| TEXAS INSTRUMENTS INCORPORATED
| Standard Linear and Logic Group
| IBIS Model of SN74LVCHR16245A
| 16-BIT BUS TRANSCEIVER WITH 3-STATE OUTPUTS
| This file contains package information for the following:
|  SSOP 48-pin (DL) package as [Component] LVCHR16245A_DL
|  TSSOP 48-pin (DGG) package as [Component] LVCHR16245A_DGG
|  VFBGA 48-pin (GQL) package as [Component] LVCHR16245A_GQL
| This device can be powered at the following Vccs:
|  1.8 volt Vcc
|  2.5 volt Vcc
|  3.3 volt Vcc
| This file provides unique models under the [Model Selector] for each Vcc.
| For operation at a specific Vcc, select the appropriate model after each
| [Model Selector] keyword.
[IBIS Ver]   3.2
[Comment char]  |_char
[File Name]   sn74lvchr16245a.ibs
[File Rev]   1.2 | e_die
[Date]   January 8, 2003
[Source]   Data created from TI-SPICE simulations at TI-SLL.
[Notes]   The following is an IBIS list for the SN74LVCHR16245A.
   Please contact sllibis@ti.com with questions and
   comments concerning SLL IBIS models.
   Non-monotonic data in ground-clamp due to bus-hold
   Non-monotonic data in pullup data due to damping resistor.
   C_comp measurement in IBIS is different than Cio in
   datasheet.
[Disclaimer] Property of Texas Instruments Incorporated. Unauthorized
   reproduction and/or distribution is strictly prohibited.
   This product is protected under copyright law.
   Created 2002, (C) Copyright 2002, Texas Instruments
   Incorporated, All Rights Reserved
   UNLESS THERE IS A SIGNED, WRITTEN AGREEMENT TO THE
   CONTRARY, TEXAS INSTRUMENTS (TI) IS PROVIDING THE IBIS
   MODELS  AND WITHOUT ANY WARRANTY, EXPRESSED OR
   IMPLIED.  TI assumes no liability for:
   1) the accuracy of the IBIS models provided to your
   company;
   2) the proper functioning of these IBIS Models in your
   design or for any resulting applications; or
   3) infringement of patents, copyrights or intellectual
   property rights resulting from your use of these IBIS
   models.
   TI provides IBIS Models as a service to our customers.
   You and your company shall not distribute, sell or give
   these models to anyone else without prior written
   permission from TI.
   TI reserves the right to make changes to our products or
   to discontinue any semiconductor product or service
   without notice, and advises our customers to obtain the
   latest version of relevant information to verify, before
   placing orders, that the information being relied on is
   current.
   Please be aware that your receipt and use of the IBIS
   information provided shall serve as acceptance of these
   terms and conditions.  If you do not accept these terms,
   you should return or destroy the IBIS models and any
   other accompanying information immediately.
| Component LVCHR16245A_DL 48-pin SSOP
[Component]   LVCHR16245A_DL
[Manufacturer]   Texas Instruments, Inc.
[Package]
|   typ   min   max
R_pkg   4.800e-02   3.800e-02   5.300e-02
L_pkg   6.046e-09   5.084e-09   7.968e-09
C_pkg   8.130e-13   5.690e-13   1.157e-12
[Pin]   signal_name   model_name   R_pin   L_pin   C_pin
1   1DIR   LVCHR16245A_DIR   4.600e-02   7.968e-09   1.017e-12
2   1B1   LVCHR16245A_IO   4.400e-02   7.299e-09   1.157e-12
3   1B2   LVCHR16245A_IO   4.300e-02   6.765e-09   1.058e-12
4   GND   GND   4.100e-02   6.269e-09   9.330e-13
5   1B3   LVCHR16245A_IO   3.800e-02   5.856e-09   8.290e-13
6   1B4   LVCHR16245A_IO   4.600e-02   5.802e-09   7.900e-13
7   VCC   POWER   5.000e-02   5.656e-09   7.380e-13
8   1B5   LVCHR16245A_IO   5.300e-02   5.500e-09   6.430e-13
9   1B6   LVCHR16245A_IO   5.200e-02   5.304e-09   6.060e-13
10   GND   GND   5.300e-02   5.189e-09   5.830e-13
11   1B7   LVCHR16245A_IO   5.100e-02   5.084e-09   5.690e-13
12   1B8   LVCHR16245A_IO   5.300e-02   5.862e-09   8.330e-13
13   2B1   LVCHR16245A_IO   5.300e-02   5.862e-09   8.330e-13
14   2B2   LVCHR16245A_IO   5.100e-02   5.084e-09   5.690e-13
15   GND   GND   5.300e-02   5.189e-09   5.830e-13
16   2B3   LVCHR16245A_IO   5.200e-02   5.304e-09   6.060e-13
17   2B4   LVCHR16245A_IO   5.300e-02   5.500e-09   6.430e-13
18   VCC   POWER   5.000e-02   5.656e-09   7.380e-13
19   2B5   LVCHR16245A_IO   4.600e-02   5.802e-09   7.900e-13
20   2B6   LVCHR16245A_IO   3.800e-02   5.856e-09   8.290e-13
21   GND   GND   4.100e-02   6.269e-09   9.330e-13
22   2B7   LVCHR16245A_IO   4.300e-02   6.765e-09   1.058e-12
23   2B8   LVCHR16245A_IO   4.400e-02   7.299e-09   1.157e-12
24   2DIR   LVCHR16245A_DIR   4.600e-02   7.968e-09   1.017e-12
25   2NOE   LVCHR16245A_NOE   4.600e-02   7.968e-09   1.017e-12
26   2A8   LVCHR16245A_IO   4.400e-02   7.299e-09   1.157e-12
27   2A7   LVCHR16245A_IO   4.300e-02   6.765e-09   1.058e-12
28   GND   GND   4.100e-02   6.269e-09   9.330e-13
29   2A6   LVCHR16245A_IO   3.800e-02   5.856e-09   8.290e-13
30   2A5   LVCHR16245A_IO   4.600e-02   5.802e-09   7.900e-13
31   VCC   POWER   5.000e-02   5.656e-09   7.380e-13
32   2A4   LVCHR16245A_IO   5.300e-02   5.500e-09   6.430e-13
33   2A3   LVCHR16245A_IO   5.200e-02   5.304e-09   6.060e-13
34   GND   GND   5.300e-02   5.189e-09   5.830e-13
35   2A2   LVCHR16245A_IO   5.100e-02   5.084e-09   5.690e-13
36   2A1   LVCHR16245A_IO   5.300e-02   5.862e-09   8.330e-13
37   1A8   LVCHR16245A_IO   5.300e-02   5.862e-09   8.330e-13
38   1A7   LVCHR16245A_IO   5.100e-02   5.084e-09   5.690e-13
39   GND   GND   5.300e-02   5.189e-09   5.830e-13
40   1A6   LVCHR16245A_IO   5.200e-02   5.304e-09   6.060e-13
41   1A5   LVCHR16245A_IO   5.300e-02   5.500e-09   6.430e-13
42   VCC   POWER   5.000e-02   5.656e-09   7.380e-13
43   1A4   LVCHR16245A_IO   4.600e-02   5.802e-09   7.900e-13
44   1A3   LVCHR16245A_IO   3.800e-02   5.856e-09   8.290e-13
45   GND   GND   4.100e-02   6.269e-09   9.330e-13
46   1A2   LVCHR16245A_IO   4.300e-02   6.765e-09   1.058e-12
47   1A1   LVCHR16245A_IO   4.400e-02   7.299e-09   1.157e-12
48   1NOE   LVCHR16245A_NOE   4.600e-02   7.967e-09   1.017e-12
| Component LVCHR16245A_DGG 48-pin TSSOP
[Component]   LVCHR16245A_DGG
[Manufacturer]   Texas Instruments, Inc.
[Package]
|   typ   min   max
R_pkg   4.400e-02   3.800e-02   5.100e-02
L_pkg   3.019e-09   2.486e-09   4.099e-09
C_pkg   5.070e-13   3.340e-13   8.090e-13
[Pin]   signal_name   model_name   R_pin   L_pin   C_pin
1   1DIR   LVCHR16245A_DIR   4.100e-02   4.017e-09   7.590e-13
2   1B1   LVCHR16245A_IO   4.200e-02   3.737e-09   7.920e-13
3   1B2   LVCHR16245A_IO   4.200e-02   3.480e-09   6.610e-13
4   GND   GND   3.800e-02   3.131e-09   5.750e-13
5   1B3   LVCHR16245A_IO   4.700e-02   3.122e-09   5.660e-13
6   1B4   LVCHR16245A_IO   4.300e-02   2.948e-09   5.040e-13
7   VCC   POWER   4.500e-02   2.845e-09   3.970e-13
8   1B5   LVCHR16245A_IO   4.900e-02   2.835e-09   3.940e-13
9   1B6   LVCHR16245A_IO   4.800e-02   2.715e-09   3.780e-13
10   GND   GND   5.000e-02   2.664e-09   3.630e-13
11   1B7   LVCHR16245A_IO   5.000e-02   2.585e-09   3.480e-13
12   1B8   LVCHR16245A_IO   4.900e-02   2.550e-09   3.370e-13
13   2B1   LVCHR16245A_IO   4.900e-02   2.541e-09   3.360e-13
14   2B2   LVCHR16245A_IO   5.000e-02   2.574e-09   3.480e-13
15   GND   GND   4.900e-02   2.618e-09   3.590e-13
16   2B3   LVCHR16245A_IO   4.600e-02   2.671e-09   3.750e-13
17   2B4   LVCHR16245A_IO   4.500e-02   2.754e-09   3.890e-13
18   VCC   POWER   4.400e-02   2.823e-09   4.500e-13
19   2B5   LVCHR16245A_IO   4.200e-02   2.968e-09   5.030e-13
20   2B6   LVCHR16245A_IO   5.100e-02   3.108e-09   5.350e-13
21   GND   GND   4.200e-02   3.175e-09   5.870e-13
22   2B7   LVCHR16245A_IO   4.100e-02   3.449e-09   6.780e-13
23   2B8   LVCHR16245A_IO   4.400e-02   3.766e-09   8.040e-13
24   2DIR   LVCHR16245A_DIR   4.300e-02   4.065e-09   7.610e-13
25   2NOE   LVCHR16245A_NOE   4.100e-02   3.994e-09   7.570e-13
26   2A8   LVCHR16245A_IO   3.900e-02   3.649e-09   7.890e-13
27   2A7   LVCHR16245A_IO   3.800e-02   3.362e-09   6.600e-13
28   GND   GND   3.800e-02   3.082e-09   5.740e-13
29   2A6   LVCHR16245A_IO   4.400e-02   2.990e-09   5.220e-13
30   2A5   LVCHR16245A_IO   4.100e-02   2.917e-09   4.950e-13
31   VCC   POWER   4.300e-02   2.820e-09   4.480e-13
32   2A4   LVCHR16245A_IO   4.300e-02   2.699e-09   3.850e-13
33   2A3   LVCHR16245A_IO   4.500e-02   2.628e-09   3.720e-13
34   GND   GND   4.600e-02   2.556e-09   3.560e-13
35   2A2   LVCHR16245A_IO   4.600e-02   2.495e-09   3.440e-13
36   2A1   LVCHR16245A_IO   4.700e-02   2.487e-09   3.340e-13
37   1A8   LVCHR16245A_IO   4.700e-02   2.490e-09   3.350e-13
38   1A7   LVCHR16245A_IO   4.600e-02   2.486e-09   3.430e-13
39   GND   GND   4.500e-02   2.566e-09   3.560e-13
40   1A6   LVCHR16245A_IO   4.400e-02   2.639e-09   3.740e-13
41   1A5   LVCHR16245A_IO   4.300e-02   2.701e-09   3.860e-13
42   VCC   POWER   4.300e-02   2.817e-09   4.500e-13
43   1A4   LVCHR16245A_IO   4.100e-02   2.935e-09   5.010e-13
44   1A3   LVCHR16245A_IO   4.700e-02   3.035e-09   5.290e-13
45   GND   GND   4.300e-02   3.171e-09   5.890e-13
46   1A2   LVCHR16245A_IO   4.000e-02   3.415e-09   6.820e-13
47   1A1   LVCHR16245A_IO   4.300e-02   3.741e-09   8.090e-13
48   1NOE   LVCHR16245A_NOE   4.400e-02   4.099e-09   7.640e-13
| Component LVCHR16245A_GQL 48-pin VFBGA
[Component]   LVCHR16245A_GQL
[Manufacturer]  Texas Instruments, Inc.
[Package]
|   typ   min   max
R_pkg   7.900e-02   4.500e-02   9.400e-02
L_pkg   2.264e-09   1.398e-09   2.722e-09
C_pkg   3.060e-13   1.170e-13   4.040e-13
[Pin]   signal_name   model_name   R_pin   L_pin   C_pin
A1   1DIR   LVCHR16245A_DIR   5.100e-02   1.531e-09   2.100e-13
B2   1B1   LVCHR16245A_IO   7.300e-02   2.572e-09   3.120e-13
B1   1B2   LVCHR16245A_IO   7.100e-02   1.835e-09   2.320e-13
B3   GND   GND   9.400e-02   2.717e-09   3.830e-13
C2   1B3   LVCHR16245A_IO   8.900e-02   2.534e-09   3.500e-13
C1   1B4   LVCHR16245A_IO   7.100e-02   1.831e-09   2.310e-13
C3   VCC   POWER   9.400e-02   2.722e-09   3.920e-13
D2   1B5   LVCHR16245A_IO   9.000e-02   2.551e-09   3.520e-13
D1   1B6   LVCHR16245A_IO   7.200e-02   1.846e-09   2.440e-13
D3   GND   GND   9.400e-02   2.719e-09   4.030e-13
E2   1B7   LVCHR16245A_IO   8.900e-02   2.541e-09   3.510e-13
E1   1B8   LVCHR16245A_IO   7.200e-02   1.850e-09   2.270e-13
F1   2B1   LVCHR16245A_IO   7.200e-02   1.850e-09   2.270e-13
F2   2B2   LVCHR16245A_IO   8.900e-02   2.541e-09   3.510e-13
G3   GND   GND   9.400e-02   2.718e-09   4.040e-13
G1   2B3   LVCHR16245A_IO   7.200e-02   1.847e-09   2.440e-13
G2   2B4   LVCHR16245A_IO   9.000e-02   2.551e-09   3.520e-13
H3   VCC   POWER   9.400e-02   2.721e-09   3.920e-13
H1   2B5   LVCHR16245A_IO   7.000e-02   1.830e-09   2.310e-13
H2   2B6   LVCHR16245A_IO   8.800e-02   2.524e-09   3.500e-13
J3   GND   GND   9.300e-02   2.709e-09   3.820e-13
J1   2B7   LVCHR16245A_IO   7.100e-02   1.851e-09   2.330e-13
J2   2B8   LVCHR16245A_IO   5.600e-02   2.605e-09   3.900e-13
K1   2DIR   LVCHR16245A_DIR   4.500e-02   1.398e-09   1.170e-13
K6   2NOE   LVCHR16245A_NOE   4.500e-02   1.512e-09   1.930e-13
J5   2A8   LVCHR16245A_IO   5.500e-02   2.492e-09   3.130e-13
J6   2A7   LVCHR16245A_IO   7.000e-02   1.821e-09   2.300e-13
J4   GND   GND   9.300e-02   2.703e-09   3.820e-13
H5   2A6   LVCHR16245A_IO   8.900e-02   2.529e-09   3.500e-13
H6   2A5   LVCHR16245A_IO   7.100e-02   1.826e-09   2.300e-13
H4   VCC   POWER   9.400e-02   2.722e-09   3.910e-13
G5   2A4   LVCHR16245A_IO   9.000e-02   2.551e-09   3.520e-13
G6   2A3   LVCHR16245A_IO   7.200e-02   1.846e-09   2.440e-13
G4   GND   GND   9.400e-02   2.719e-09   4.040e-13
F5   2A2   LVCHR16245A_IO   8.800e-02   2.510e-09   3.490e-13
F6   2A1   LVCHR16245A_IO   7.200e-02   1.850e-09   2.270e-13
E6   1A8   LVCHR16245A_IO   7.100e-02   1.850e-09   2.270e-13
E5   1A7   LVCHR16245A_IO   8.900e-02   2.529e-09   3.500e-13
D4   GND   GND   9.400e-02   2.719e-09   4.030e-13
D6   1A6   LVCHR16245A_IO   7.200e-02   1.847e-09   2.430e-13
D5   1A5   LVCHR16245A_IO   8.900e-02   2.550e-09   3.520e-13
C4   VCC   POWER   9.400e-02   2.722e-09   3.910e-13
C6   1A4   LVCHR16245A_IO   7.100e-02   1.827e-09   2.300e-13
C5   1A3   LVCHR16245A_IO   8.900e-02   2.539e-09   3.500e-13
B4   GND   GND   9.300e-02   2.705e-09   3.820e-13
B6   1A2   LVCHR16245A_IO   7.100e-02   1.831e-09   2.270e-13
B5   1A1   LVCHR16245A_IO   7.300e-02   2.685e-09   3.800e-13
A6   1NOE   LVCHR16245A_NOE   5.100e-02   1.417e-09   1.330e-13
| Model LVCHR16245A_DIR
[Model Selector]   LVCHR16245A_DIR
LVCHR16245A_DIR_18   1.8 volt Vcc
LVCHR16245A_DIR_25   2.5 volt Vcc
LVCHR16245A_DIR_33   3.3 volt Vcc
| Model LVCHR16245A_NOE
[Model Selector]   LVCHR16245A_NOE
LVCHR16245A_NOE_18   1.8 volt Vcc
LVCHR16245A_NOE_25   2.5 volt Vcc
LVCHR16245A_NOE_33   3.3 volt Vcc
| Model LVCHR16245A_IO
[Model Selector]   LVCHR16245A_IO
LVCHR16245A_IO_18   1.8 volt Vcc
LVCHR16245A_IO_25   2.5 volt Vcc
LVCHR16245A_IO_33   3.3 volt Vcc
| Models and submodels in the file (9): LVCHR16245A_DIR_18 (Input), LVCHR16245A_DIR_25 (Input), LVCHR16245A_DIR_33 (Input), LVCHR16245A_NOE_18 (Input), LVCHR16245A_NOE_25 (Input), LVCHR16245A_NOE_33 (Input), LVCHR16245A_IO_18 (I/O), LVCHR16245A_IO_25 (I/O), LVCHR16245A_IO_33 (I/O)
